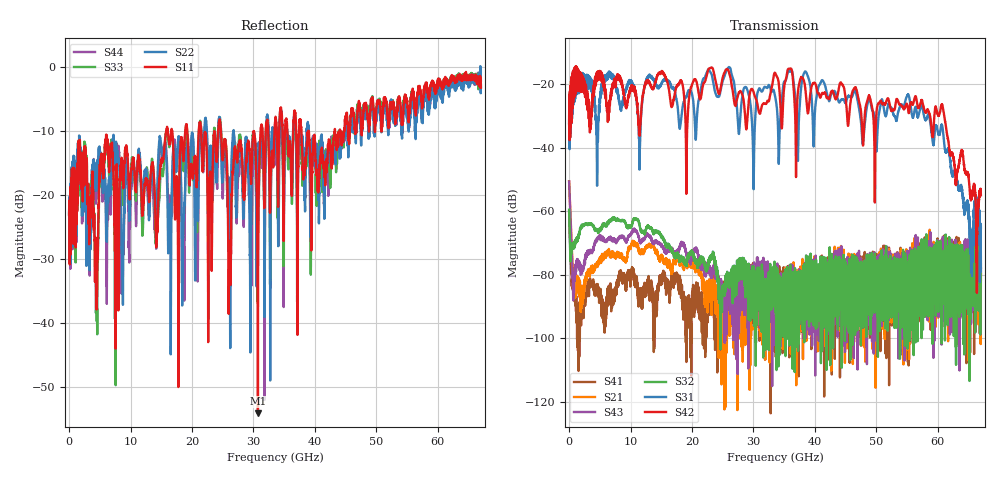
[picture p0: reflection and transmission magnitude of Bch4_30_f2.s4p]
!Agilent Technologies,N5247A,US51170199,A.09.90.13
!Agilent N5247A: A.09.90.13
!Date: Thursday, October 18, 2018 10:15:21
!Correction: S11(Full 4 Port(1,2,3,4))
!S12(Full 4 Port(1,2,3,4))
!S13(Full 4 Port(1,2,3,4))
!S14(Full 4 Port(1,2,3,4))
!S21(Full 4 Port(1,2,3,4))
!S22(Full 4 Port(1,2,3,4))
!S23(Full 4 Port(1,2,3,4))
!S24(Full 4 Port(1,2,3,4))
!S31(Full 4 Port(1,2,3,4))
!S32(Full 4 Port(1,2,3,4))
!S33(Full 4 Port(1,2,3,4))
!S34(Full 4 Port(1,2,3,4))
!S41(Full 4 Port(1,2,3,4))
!S42(Full 4 Port(1,2,3,4))
!S43(Full 4 Port(1,2,3,4))
!S44(Full 4 Port(1,2,3,4))
!S4P File: Measurements: <S11,S12,S13,S14>,
!<S21,S22,S23,S24>,
!<S31,S32,S33,S34>,
!<S41,S42,S43,S44>:
# Hz S  dB  R 50
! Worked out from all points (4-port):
!   6701 points, 10 MHz to 67 GHz, reference 50 ohm
!   strongest paths, dB at 10 MHz, 16.76 GHz, 33.51 GHz, 50.25 GHz, 67 GHz:
!     S42: -32.2, -26.8, -16.4, -26.3, -54.9
!     S31: -32.6, -21.2, -23.7, -32.3, -65.3
!     S32: -59.5, -72.2, -90.0, -77.7, -77.7
!     S43: -50.6, -72.2, -80.2, -82.9, -80.1
!     S21: -50.6, -78.8, -85.5, -81.0, -79.8
!     S41: -60.1, -81.2, -86.7, -75.0, -78.0
!   lowest |S11| = -54.1 dB at 30.73 GHz (marker M1), VSWR 1.00, Z = 50 + j0.198 ohm
!   |S11| at or under -10 dB: start of sweep to 15.79 GHz; 24.7 GHz to 30.02 GHz (5.321 GHz wide, 19.4 % of centre); 38.96 GHz to 43.22 GHz (4.262 GHz wide, 10.4 % of centre)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
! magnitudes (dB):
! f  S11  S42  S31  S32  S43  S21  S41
! 10 MHz  -23.0  -32.2  -32.6  -59.5  -50.6  -50.6  -60.1
! 969.9 MHz  -23.6  -21.4  -19.1  -70.5  -77.8  -81.6  -84.8
! 4.519 GHz  -37.0  -16.5  -41.8  -65.9  -68.8  -76.9  -84.3
! 6.039 GHz  -10.5  -25.9  -17.2  -64.5  -69.4  -72.8  -91.6
! 30.73 GHz  -54.1  -27.3  -22.3  -79.9  -78.1  -78.9  -79.5
! 55.12 GHz  -6.4  -27.6  -23.3  -79.2  -81.9  -73.1  -76.0
! 67 GHz  -3.2  -54.9  -65.3  -77.7  -80.1  -79.8  -78.0
